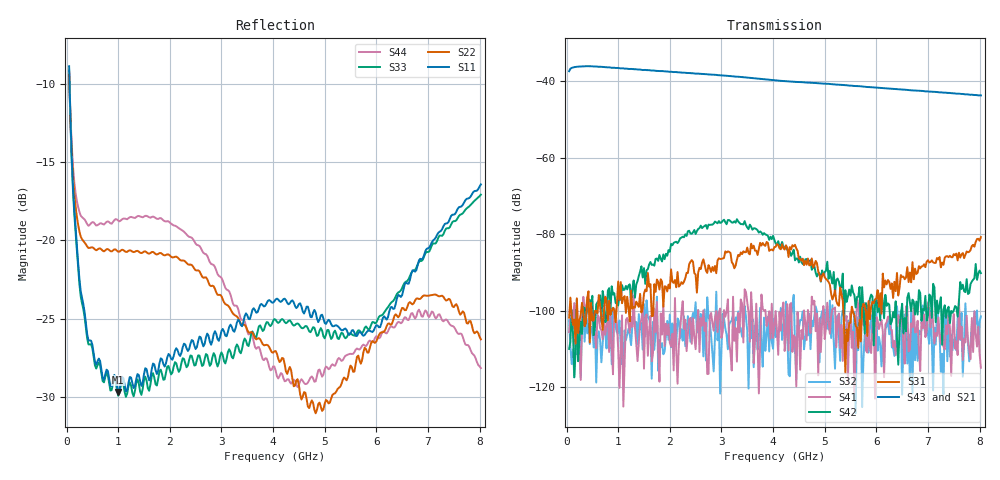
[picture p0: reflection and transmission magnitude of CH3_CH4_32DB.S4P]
!Agilent Technologies,E5071C,MY46316741,A.11.02
!Date: Thu May 28 15:01:45 2026
!Data & Calibration Information:
!1:CH3 INPUT 2:CH3 OUTPUT 3:CH4 INPUT 4:CH4 OUTPUT
!Freq	S11:SOLT4(ON)	S12:SOLT4(ON)	S13:SOLT4(ON)	S14:SOLT4(ON)
!	S21:SOLT4(ON)	S22:SOLT4(ON)	S23:SOLT4(ON)	S24:SOLT4(ON)
!	S31:SOLT4(ON)	S32:SOLT4(ON)	S33:SOLT4(ON)	S34:SOLT4(ON)
!	S41:SOLT4(ON)	S42:SOLT4(ON)	S43:SOLT4(ON)	S44:SOLT4(ON)
!PortZ  Port1:50+j0  Port2:50+j0  Port3:50+j0  Port4:50+j0
!Above PortZ is port z conversion or system Z0 setting when saving the data.
!When reading, reference impedance value at option line is always used.
# Hz S dB R 50
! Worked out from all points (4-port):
!   320 points, 50 MHz to 8.025 GHz, reference 50 ohm
!   strongest paths, dB at 50 MHz, 2.05 GHz, 4.05 GHz, 6.05 GHz, 8.025 GHz:
!     S43: -37.4, -37.6, -39.8, -41.7, -43.7
!     S21: -37.5, -37.6, -39.8, -41.7, -43.6
!     S31: -101.8, -92.4, -83.3, -99.0, -80.7
!     S42: -110.0, -82.9, -82.4, -97.0, -90.2
!     S41: -105.6, -106.0, -100.1, -104.8, -114.9
!     S32: -102.5, -103.3, -106.9, -106.8, -101.4
!   lowest |S11| = -29.7 dB at 1 GHz (marker M1), VSWR 1.07, Z = 48 - j2.51 ohm
!   |S11| at or under -10 dB: 58.58 MHz to end of sweep
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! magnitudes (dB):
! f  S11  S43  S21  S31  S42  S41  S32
! 50 MHz  -8.9  -37.4  -37.5  -101.8  -110.0  -105.6  -102.5
! 275 MHz  -23.3  -36.2  -36.2  -100.9  -102.8  -118.1  -117.5
! 1 GHz  -29.7  -36.5  -36.6  -92.3  -98.6  -109.9  -105.8
! 3.3 GHz  -25.3  -38.8  -38.9  -86.6  -76.1  -113.3  -102.4
! 4.825 GHz  -24.6  -40.5  -40.5  -87.0  -90.0  -105.3  -98.8
! 6.775 GHz  -21.9  -42.4  -42.4  -90.4  -97.6  -105.6  -105.9
! 8.025 GHz  -16.4  -43.7  -43.6  -80.7  -90.2  -114.9  -101.4
